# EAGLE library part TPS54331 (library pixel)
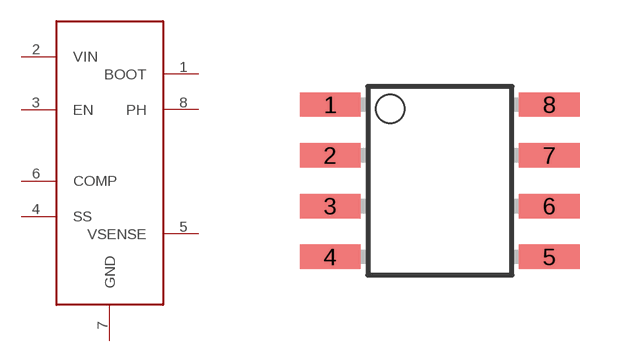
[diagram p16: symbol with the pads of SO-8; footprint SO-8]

Designator prefix -

## TPS54331  [SO-8]
1  BOOT
2  VIN
3  EN
4  SS
5  VSENSE
6  COMP
7  GND
8  PH

## Footprint SO-8 (pad centres in mm)
SO 8 small outline
smd 1.524 x 0.61: 1 -2.743,1.905; 2 -2.743,0.635; 3 -2.743,-0.635; 4 -2.743,-1.905; 5 2.743,-1.905; 6 2.743,-0.635; 7 2.743,0.635; 8 2.743,1.905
